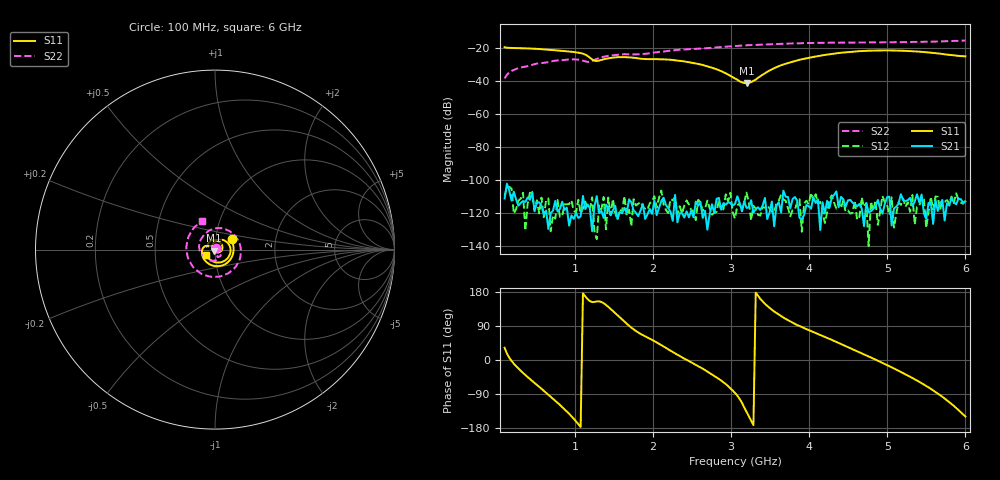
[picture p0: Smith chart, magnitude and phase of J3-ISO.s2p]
!Agilent Technologies,E8364B,MY43040379,A.07.50.67
!Agilent E8364B: A.07.50.67
!Date: Tuesday, March 24, 2026 11:37:38
!Correction: S11(Full 2 Port(1,2))
!S21(Full 2 Port(1,2))
!S12(Full 2 Port(1,2))
!S22(Full 2 Port(1,2))
!S2P File: Measurements: S11, S21, S12, S22:
# Hz S  dB  R 50
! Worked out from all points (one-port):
!   201 points, 100 MHz to 6 GHz, reference 50 ohm
!   lowest |S11| = -41.1 dB at 3.197 GHz (marker M1), VSWR 1.02, Z = 49.4 - j0.598 ohm
!   |S11| at or under -10 dB: start of sweep to end of sweep
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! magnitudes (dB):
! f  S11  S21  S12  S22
! 100 MHz  -19.3  -111.4  -110.1  -38.2
! 129.5 MHz  -19.6  -102.3  -104.3  -36.0
! 188.5 MHz  -19.7  -112.6  -105.2  -33.7
! 513 MHz  -20.3  -113.6  -112.5  -29.2
! 926 MHz  -21.9  -127.9  -114.7  -26.7
! 1.103 GHz  -23.2  -109.8  -117.3  -27.5
! 1.192 GHz  -25.6  -117.2  -118.2  -28.1
! 1.28 GHz  -27.7  -109.9  -136.1  -26.3
! 1.546 GHz  -25.3  -123.8  -124.2  -23.9
! 2.076 GHz  -26.6  -117.1  -111.1  -22.2
! 2.372 GHz  -27.7  -120.2  -120.4  -20.7
! 2.637 GHz  -30.0  -123.1  -118.9  -20.0
! 2.844 GHz  -33.2  -111.0  -112.3  -19.2
! 3.05 GHz  -38.2  -114.6  -123.5  -18.5
! 3.197 GHz  -41.1  -117.1  -107.7  -18.1
! 3.256 GHz  -40.5  -112.4  -124.6  -17.9
! 3.493 GHz  -33.4  -119.9  -117.6  -17.5
! 3.64 GHz  -30.2  -120.0  -109.0  -17.3
! 4.053 GHz  -25.2  -110.6  -112.6  -16.6
! 4.525 GHz  -22.0  -112.1  -120.5  -16.5
! 5.027 GHz  -21.2  -110.2  -121.3  -16.3
! 6 GHz  -24.8  -113.1  -112.7  -15.1
